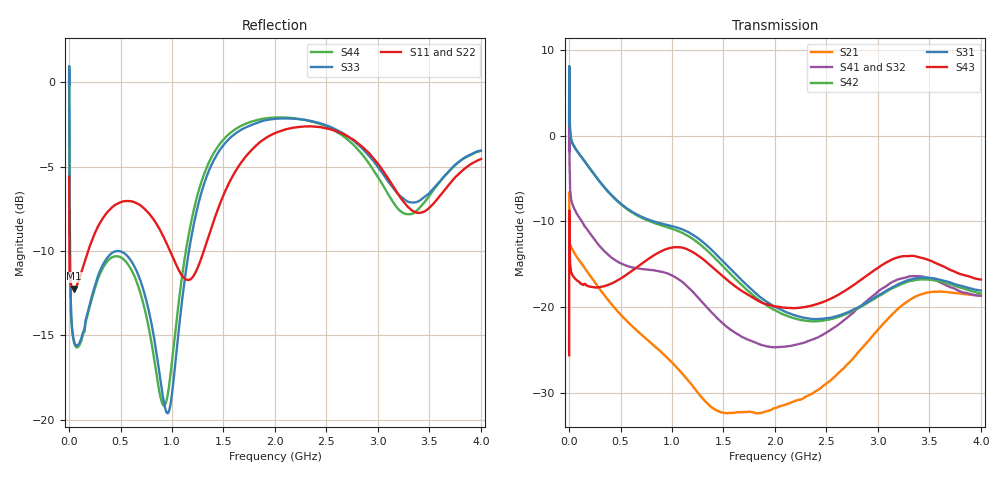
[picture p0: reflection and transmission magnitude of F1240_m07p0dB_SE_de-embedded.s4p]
! Integrated Device Technology
! Corporate Headquarters
! 6024 Silver Creek Valley Road
! San Jose, CA 95138  USA
! Phone:  1-408-284-8200
! Toll Free:  1-800-223-1366
! Webpage:  http://www.idt.com/
! Timing and RF Division
! 515 Groton Road, Suite 102
! Westford, MA 01886-6024
! Device:  F1240
! Description: Dual Intermediate Frequency Digital Variable Gain Amplifier
! Frequency:  10.0 -  500.00 MHz
! Package:  5x5 mm QFN Plastic Package: 32 pin
! Ports:  8 RF, 20 DC
!  Pin  1  = GA3 / Data  Pin 17  = RF OUT_B+
!  Pin  2  = GA4 / CLK  Pin 18  = RF OUT_B-
!  Pin  3  = GA5  Pin 19  = STBY_B
!  Pin  4  = VMODE  Pin 20  = Ground
!  Pin  5  = No Connect  Pin 21  = Ground
!  Pin  6  = GB5  Pin 22  = STB_A
!  Pin  7  = GB4  Pin 23  = RF OUT_A-  = Port 4
!  Pin  8  = GB3  Pin 24  = RF OUT_A+  = Port 3
!  Pin  9  = GB2  Pin 25  = GA0
!  Pin 10  = GB1  Pin 26  = ISET_A
!  Pin 11  = RF IN_B+  Pin 27  = VCC
!  Pin 12  = RF IN_B-  Pin 28  = Ground
!  Pin 13  = Ground  Pin 29  = RF IN_A-  = Port 2
!  Pin 14  = VCC  Pin 30  = RF IN_A+  = Port 1
!  Pin 15  = ISET_B  Pin 31  = GA1
!  Pin 16  = GB0  Pin 32  = GA2 / CSb
! Gain  = +19.5 dB
! State  = 1
! Voltage  = +5.00 V
! Current  = 85.292 mA (one channel only)
! Temperture  =  +25 C
! Test Date  =  2017-10-18
! Board  =  EB4031
! Data:  The device was measured on a custom evaluation board which has
!  individual transmission lines to the RF pins.  Data was collected
!  using a calibrated network analyzer.  The evaluation board was
!  de-embedded using Automatic Fixture Removal.
!  The reference plane is the edge of the package pin.
!  Only Channel A was measured.
!  This data is in single-ended operation.  If your needs are balanced
!  or differential S-parameters then this file needs to be used a
!  linear simulator.
! File Date:  2017-11-10  MJV
! Note:
!  Integrated Device Technology supplies this data as a sample of measured
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# Hz S dB R 100
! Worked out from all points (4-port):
!   410 points, 500 kHz to 4 GHz, reference 100 ohm
!   strongest paths, dB at 500 kHz, 930 MHz, 1.96 GHz, 2.98 GHz, 4 GHz:
!     S43: -25.6, -13.3, -19.8, -15.6, -16.8
!     S31: 1.3, -10.3, -19.7, -18.8, -18.1
!     S42: 1.3, -10.6, -20.1, -18.9, -18.4
!     S41: -1.8, -16.0, -24.6, -18.4, -18.7
!     S32: -1.8, -16.2, -24.5, -18.7, -19.0
!     S21: -6.6, -25.6, -32.0, -22.9, -18.7
!   lowest |S11| = -12.2 dB at 50 MHz (marker M1), VSWR 1.65, Z = 138 - j45.4 ohm
!   |S11| at or under -10 dB: 2.944 MHz to 184.7 MHz (181.8 MHz wide, 194 % of centre); 980.4 MHz to 1.308 GHz (327.9 MHz wide, 28.7 % of centre)
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500000  -5.61 -5.6  -6.60 -5.8  -31.42 78.2  -34.60 77.1
        -6.61 -5.8  -5.61 -5.6  -34.57 75.9  -31.39 79.3
        1.26 -110.3  -1.76 -112.2  -0.15 0.1  -25.61 -38.5
        -1.78 -111.1  1.26 -109.2  -25.61 -38.5  -0.16 2.4
2000000  -8.25 -29.1  -9.57 -29.5  -23.13 21.2  -26.97 5.1
         -9.57 -29.5  -8.22 -29.1  -26.93 4.8  -23.11 21.5
         7.41 176.2  3.80 161.4  -0.40 -53.4  -8.70 -143.5
         3.76 161.7  7.41 176.5  -8.70 -143.5  -0.44 -53.1
4000000  -10.85 -22.4  -12.09 -19.3  -23.91 5.0  -30.02 -12.3
         -12.09 -19.3  -10.85 -22.7  -29.99 -12.5  -23.91 5.2
         3.87 156.3  -1.76 140.5  -4.90 -85.6  -11.36 174.7
         -1.80 140.7  3.88 156.5  -11.36 174.6  -4.95 -85.6
5e7  -12.23 -39.2  -13.64 -23.4  -25.08 -17.1  -32.82 -20.0
     -13.65 -23.4  -12.19 -39.8  -32.83 -19.9  -25.05 -17.1
     -1.29 152.3  -8.50 142.9  -15.38 -160.1  -16.59 153.5
     -8.49 143.0  -1.24 152.1  -16.55 153.4  -15.45 -160.7
5.2e8  -7.07 -148.1  -21.12 -128.3  -28.60 -104.7  -36.68 -90.9
       -21.11 -128.2  -7.03 -149.0  -36.82 -88.7  -28.89 -104.8
       -8.09 25.4  -15.09 -23.3  -10.07 -173.5  -16.60 10.9
       -14.99 -24.6  -8.16 23.8  -16.52 10.7  -10.44 -174.2
2.91e9  -4.18 101.1  -23.93 -29.5  -28.28 -157.9  -30.55 -143.4
        -23.91 -29.6  -3.97 101.8  -31.15 -130.2  -29.71 -150.6
        -19.33 -72.3  -19.40 -153.4  -4.34 94.0  -16.96 -91.8
        -19.10 -165.0  -19.43 -69.0  -16.16 -89.7  -4.79 86.6
4e9  -4.56 -127.7  -18.66 118.8  -27.19 -28.6  -28.22 -13.3
     -18.65 118.7  -4.30 -126.5  -28.78 0.9  -29.08 -19.0
     -18.06 50.7  -19.01 -46.1  -4.05 -133.3  -18.20 62.4
     -18.66 -60.5  -18.40 56.8  -16.77 55.8  -4.07 -143.2
